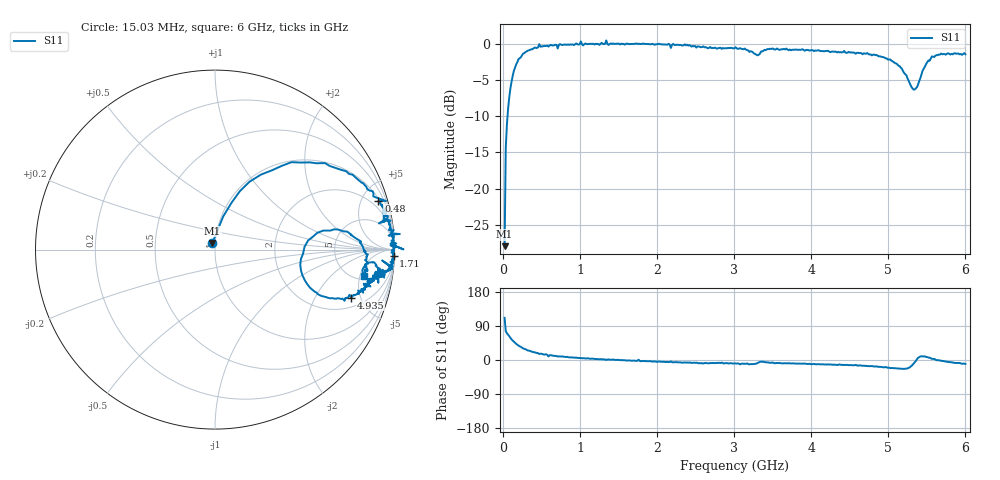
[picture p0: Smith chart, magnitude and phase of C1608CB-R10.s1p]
!	Network	Analyzer	HP8753E.07.74:	Oct	30	2002	Serial	No.	JP38451487
!	Hewlett-Packard
!	7	Sep	2009	9:53:08
!	Frequency	S11
#	HZ	S	RI	R	50
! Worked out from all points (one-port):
!   400 points, 15.03 MHz to 6 GHz, reference 50 ohm
!   lowest |S11| = -27.9 dB at 15.03 MHz (marker M1), VSWR 1.08, Z = 48.4 + j3.63 ohm
!   |S11| at or under -10 dB: start of sweep to 53.12 MHz
!   S11 on the Smith chart (normalised r, x): 15.03 MHz: 0.97, +0.07; 480 MHz: 1.19, +6.63; 1.71 GHz: 8, -59; 4.935 GHz: 2.72, -4.14; 6 GHz: 5.70, -5.87
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1.502992e7  -0.0146 0.0374
3.002985e7  0.0459 0.185
6.00297e7  0.139 0.326
1.050295e8  0.318 0.442
2.550287e8  0.732 0.436
4.800276e8  0.91 0.272
5.550272e8  0.93 0.25
5.850271e8  0.94 0.154
6.150269e8  0.955 0.215
7.650262e8  0.963 0.163
1.245024e9  0.978 0.0323
1.335023e9  1.05 0.00122
1.365023e9  0.978 0.0241
1.515022e9  0.985 -0.0036
1.710021e9  0.995 -0.0329
2.265019e9  0.976 -0.102
3.015015e9  0.931 -0.152
3.300014e9  0.821 -0.114
3.435013e9  0.911 -0.101
3.765011e9  0.895 -0.138
4.515007e9  0.847 -0.201
4.935005e9  0.76 -0.267
5.265004e9  0.515 -0.194
5.370003e9  0.499 0.016
5.460003e9  0.664 0.113
5.565002e9  0.814 0.0448
5.685002e9  0.852 -0.0273
6e9  0.831 -0.148
